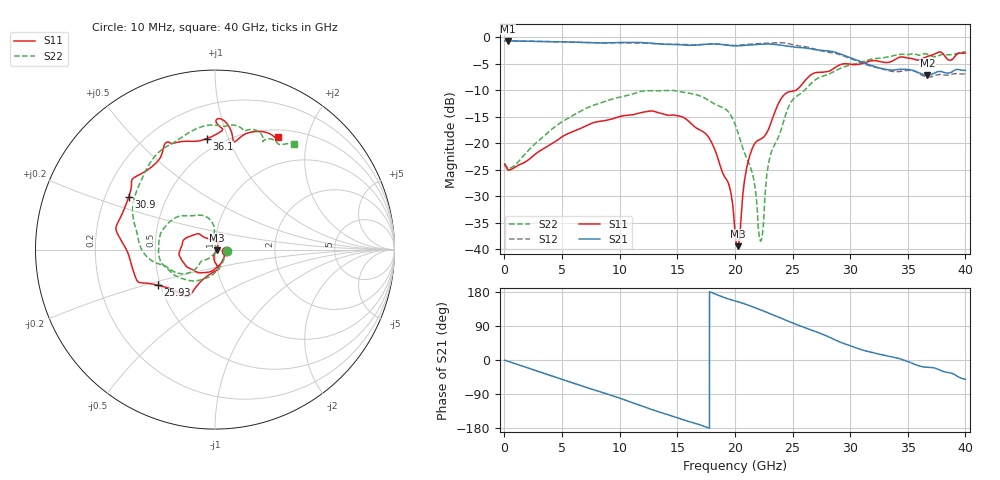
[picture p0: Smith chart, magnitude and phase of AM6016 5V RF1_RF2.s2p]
!Agilent Technologies,E8364B,MY43040894,A.07.50.67
!Agilent E8364B: A.07.50.67
!Date: Thursday, January 16, 2020 10:45:04
!Correction: S11(Full 2 Port(1,2))
!S21(Full 2 Port(1,2))
!S12(Full 2 Port(1,2))
!S22(Full 2 Port(1,2))
!S2P File: Measurements: S11, S21, S12, S22:
# Hz S  dB  R 50
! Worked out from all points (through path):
!   6401 points, 10 MHz to 40 GHz, reference 50 ohm
!   highest |S21| = -0.64 dB at 291.2 MHz (marker M1); lowest = -7.2 dB at 36.7 GHz (marker M2)
!   group delay of S21, straight-line fit = 29.2 ps
!   lowest |S11| = -39.4 dB at 20.23 GHz (marker M3), VSWR 1.02, Z = 51 - j0.454 ohm
!   |S11| at or under -10 dB: start of sweep to 25.26 GHz
!   |S22| runs from -38.5 to -2.7 dB; largest |S21 - S12| = 0.055
!   S11 on the Smith chart (normalised r, x): 10 MHz: 1.14, -0.01; 25.93 GHz: 0.49, -0.22; 30.9 GHz: 0.30, +0.26; 36.1 GHz: 0.42, +0.84; 40 GHz: 0.60, +1.53
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1e7  -23.93 -5.7  -0.66 -0.7  -0.56 -1.0  -23.78 -5.5
2.911797e8  -24.98 -7.4  -0.64 -3.1  -0.63 -3.2  -24.75 -11.9
6.677083e9  -17.10 -113.9  -0.93 -68.0  -0.92 -67.9  -13.81 -121.4
1.035116e10  -14.75 -147.6  -0.95 -104.3  -1.03 -104.5  -11.10 -154.6
1.334417e10  -14.18 -178.0  -1.19 -136.4  -1.21 -135.5  -10.09 176.1
1.773682e10  -18.91 134.1  -1.24 -179.4  -1.29 -179.2  -11.93 131.8
1.949888e10  -27.95 65.9  -1.51 160.3  -1.45 161.5  -14.22 106.7
2.0005e10  -36.80 33.2  -1.59 155.9  -1.50 156.7  -16.35 95.9
2.022994e10  -39.39 -24.5  -1.59 154.0  -1.48 154.6  -17.74 92.6
2.107973e10  -24.02 -92.9  -1.45 145.7  -1.31 146.1  -23.05 98.1
2.164834e10  -20.27 -80.2  -1.38 139.3  -1.23 140.1  -26.99 94.6
2.224819e10  -19.14 -79.1  -1.28 132.1  -1.14 132.9  -38.41 -4.6
2.311672e10  -16.19 -106.9  -1.26 121.3  -1.05 121.7  -21.93 -134.3
2.475381e10  -10.21 -122.7  -1.70 100.5  -1.22 99.1  -12.63 -145.0
2.593477e10  -8.55 -148.0  -1.95 86.9  -1.70 84.2  -10.18 -164.2
2.667208e10  -6.94 -155.7  -2.19 78.5  -2.04 74.6  -8.54 -172.7
3.090228e10  -4.99 148.8  -4.54 28.1  -4.70 26.6  -4.70 132.1
3.333917e10  -4.69 124.7  -6.11 10.0  -6.28 7.8  -3.66 105.6
3.610098e10  -4.15 94.3  -6.77 -16.4  -6.98 -18.3  -3.30 75.5
3.670082e10  -3.58 86.8  -7.17 -19.0  -7.43 -22.1  -3.15 68.7
3.87878e10  -4.24 79.2  -6.54 -34.8  -6.95 -37.4  -3.23 58.2
4e10  -2.91 60.9  -6.21 -51.1  -6.89 -52.9  -2.67 53.3
